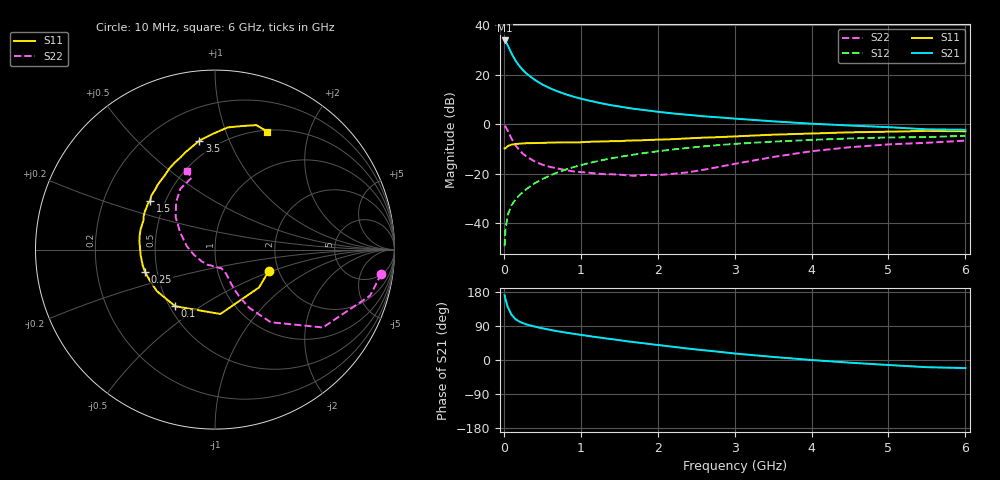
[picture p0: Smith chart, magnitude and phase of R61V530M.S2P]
! SIEMENS Small Signal Semiconductors
! BFR193
! Si NPN RF Bipolar Junction Transistor in SOT23
! VCE = 1.5 V  IC = 30 mA
! Common Emitter S-Parameters:  May  1996
# GHz  S  MA  R  50
!  f  S11  S21  S12  S22
! GHz  MAG  ANG  MAG  ANG  MAG  ANG  MAG  ANG
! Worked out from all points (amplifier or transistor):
!   36 points, 10 MHz to 6 GHz, reference 50 ohm
!   highest |S21| = 33.9 dB at 10 MHz (marker M1)
!   |S21| within 3 dB of that: start of sweep to 66.06 MHz
!   unconditionally stable (mu >= 1): 434.4 MHz to 2.032 GHz
!   at 250 MHz: K = 0.92, MSG = 24.6 dB, |S12| = -27.4 dB
!   at 1.4 GHz: K = 1.02, MAG = 9.8 dB, |S12| = -13.8 dB
!   at 6 GHz: K = 0.96, MSG = 1.2 dB, |S12| = -4.7 dB
!   S11 on the Smith chart (normalised r, x): 10 MHz: 1.78, -0.47; 100 MHz: 0.54, -0.40; 250 MHz: 0.43, -0.13; 1.5 GHz: 0.41, +0.28; 3.5 GHz: 0.40, +0.78; 6 GHz: 0.52, +1.41
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0.01  0.3228 -21.5  49.51 170.6  0.0034 80.6  0.9362 -8.3
0.02  0.3237 -40.6  48.1 161.4  0.0069 81.4  0.9016 -16.5
0.05  0.3599 -85.2  39.66 140.1  0.0146 68.4  0.7416 -35.8
0.1  0.3856 -125.0  27 119.5  0.0228 64.4  0.5104 -52.5
0.15  0.3981 -144.4  19.58 108.2  0.0297 64.8  0.3769 -59.5
0.2  0.4019 -154.4  15.23 101.7  0.0362 67.2  0.3012 -62.5
0.25  0.409 -162.1  12.35 97.0  0.0427 68.3  0.2508 -63.9
0.3  0.4125 -167.7  10.4 93.5  0.0495 69.9  0.2185 -64.6
0.4  0.4155 -175.7  7.934 88.2  0.0635 71.1  0.1769 -64.8
0.5  0.418 178.6  6.366 83.7  0.0775 71.6  0.1515 -65.2
0.6  0.4237 173.7  5.347 79.6  0.0916 71.1  0.1368 -66.0
0.7  0.4269 169.2  4.615 75.8  0.1058 70.4  0.1269 -67.6
0.8  0.4294 165.3  4.056 72.5  0.12 69.5  0.1182 -69.4
0.9  0.4292 162.1  3.629 69.3  0.1343 68.6  0.1109 -70.8
1.1  0.4398 154.5  3.023 63.4  0.1622 66.3  0.1046 -77.3
1.5  0.4519 143.1  2.289 52.4  0.2174 60.8  0.0954 -94.0
2.2  0.4977 124.5  1.65 34.9  0.3083 50.3  0.0991 -138.2
3  0.5658 107.1  1.298 17.2  0.3996 37.5  0.1574 173.5
3.5  0.6137 98.1  1.143 8.1  0.4436 29.5  0.2168 153.7
4.5  0.6846 84.0  0.94 -7.1  0.5148 15.2  0.3422 129.3
5.5  0.7309 71.6  0.787 -19.0  0.5478 1.4  0.4203 108.1
6  0.7187 66.1  0.771 -21.3  0.5818 -2.7  0.465 109.7
